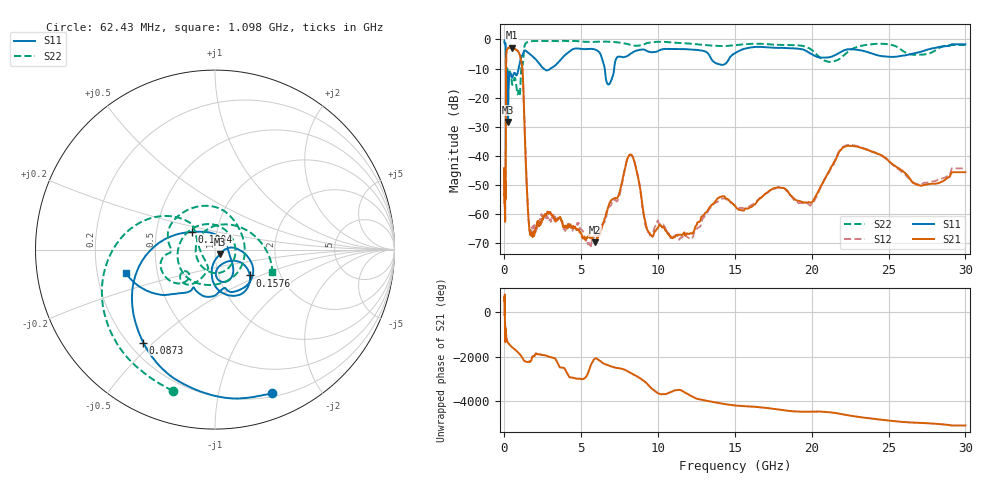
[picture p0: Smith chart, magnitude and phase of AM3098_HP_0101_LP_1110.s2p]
! Date/Time: Thu, Feb 28, 2019 8:37 AM
! Network Analyzer: Agilent Technologies E8364B Rev: A.07.50.67
! Sweep from 0.010 to 30.000 GHz, 1601 Points, Sweep Type: LOG
! Power Supply: 5.022 V, 0.002 A
# Hz S DB R 50
!freq MagS11 AngS11 MagS21 AngS21 MagS12 AngS12 MagS22 AngS22
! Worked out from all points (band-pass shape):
!   1601 points, 10 MHz to 30 GHz, reference 50 ohm
!   highest |S21| = -2.79 dB at 493.1 MHz (marker M1); lowest = -69.7 dB at 5.9 GHz (marker M2)
!   |S21| within 3 dB of the highest: 114.7 MHz to 1.028 GHz (913.2 MHz wide, 160 % of centre)
!   lowest |S11| = -28.4 dB at 236.3 MHz (marker M3), VSWR 1.08, Z = 52.9 - j2.61 ohm
!   |S11| at or under -10 dB: 97.45 MHz to 922.7 MHz (825.2 MHz wide, 162 % of centre); 2.531 GHz to 2.997 GHz (466.2 MHz wide, 16.9 % of centre); 6.525 GHz to 7.142 GHz (617.5 MHz wide, 9.04 % of centre)
!   |S22| runs from -22.2 to -0.5 dB; largest |S21 - S12| = 0.011
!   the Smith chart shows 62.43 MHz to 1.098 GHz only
!   S11 on the Smith chart (normalised r, x): 62.43 MHz: 0.23, -1.44; 87.3 MHz: 0.26, -0.47; 100.4 MHz: 0.76, +0.15; 157.6 MHz: 1.40, -0.43; 1.098 GHz: 0.33, -0.12
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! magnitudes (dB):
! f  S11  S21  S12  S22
! 10 MHz  -0.3  -44.2  -46.3  -0.6
! 38.04 MHz  -0.5  -59.7  -57.5  -1.0
! 62.43 MHz  -1.3  -53.2  -51.5  -1.7
! 87.3 MHz  -3.7  -39.5  -38.8  -4.1
! 100.4 MHz  -15.8  -13.3  -13.3  -20.1
! 144.7 MHz  -17.4  -3.7  -3.7  -13.7
! 157.6 MHz  -12.3  -3.5  -3.5  -11.5
! 236.3 MHz  -28.4  -2.9  -2.9  -12.0
! 309.6 MHz  -12.7  -2.9  -2.8  -11.3
! 493.1 MHz  -13.1  -2.8  -2.8  -15.3
! 550.5 MHz  -12.5  -3.0  -2.9  -15.1
! 1.098 GHz  -5.8  -7.6  -7.6  -9.3
! 1.606 GHz  -4.8  -64.5  -64.1  -0.8
! 2.084 GHz  -7.1  -64.4  -65.5  -0.5
! 5.9 GHz  -3.5  -69.7  -67.2  -0.8
! 6.821 GHz  -15.4  -56.5  -57.4  -0.8
! 7.926 GHz  -5.9  -42.5  -42.2  -1.5
! 9.443 GHz  -4.3  -66.5  -66.8  -1.1
! 11.19 GHz  -3.3  -67.2  -67.4  -1.2
! 19.61 GHz  -3.9  -56.0  -56.4  -2.5
! 22.67 GHz  -3.4  -36.6  -36.3  -3.2
! 30 GHz  -1.7  -45.6  -44.3  -1.9
